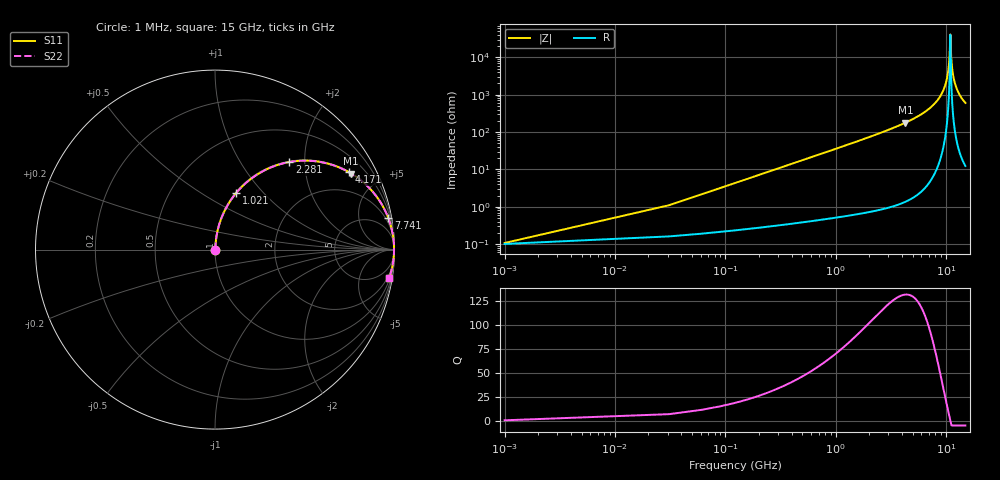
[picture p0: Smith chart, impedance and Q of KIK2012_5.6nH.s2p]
!version-2
!date-01.2022
!Series
# MHz S RI R 50
!Freq ReS11 ImS11 ReS21 ImS21 ReS12 ImS12 ReS22 ImS22
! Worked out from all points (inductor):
!   501 points, 1 MHz to 15 GHz, reference 50 ohm
!   read as one part in series: L = 5.6 nH near 61 MHz
!   highest Q = 131 at 4.291 GHz (marker M1), where L = 6.61 nH
!   self-resonance near 10.95 GHz
!   S11 on the Smith chart (normalised r, x): 1 MHz: 1.00, +0.00; 1.021 GHz: 1.01, +0.72; 2.281 GHz: 1.02, +1.68; 4.171 GHz: 1.03, +3.43; 7.741 GHz: 1, +11; 15 GHz: 1, -12
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1  0.00101 0.000351  0.999 -0.000351  0.999 -0.000351  0.00101 0.000351
91  0.00315 0.0319  0.9969 -0.0319  0.9969 -0.0319  0.00315 0.0319
211  0.00822 0.0735  0.9918 -0.0735  0.9918 -0.0735  0.00822 0.0735
511  0.0349 0.1732  0.9651 -0.1732  0.9651 -0.1732  0.0349 0.1732
1021  0.1196 0.3174  0.8804 -0.3174  0.8804 -0.3174  0.1196 0.3174
2281  0.4139 0.4879  0.5861 -0.4879  0.5861 -0.4879  0.4139 0.4879
2521  0.4676 0.4945  0.5324 -0.4945  0.5324 -0.4945  0.4676 0.4945
4171  0.7449 0.4321  0.2551 -0.4321  0.2551 -0.4321  0.7449 0.4321
4291  0.7591 0.4239  0.2409 -0.4239  0.2409 -0.4239  0.7591 0.4239
5011  0.8306 0.3713  0.1694 -0.3713  0.1694 -0.3713  0.8306 0.3713
7501  0.9589 0.1927  0.0411 -0.1927  0.0411 -0.1927  0.9589 0.1927
7741  0.9652 0.1771  0.0348 -0.1771  0.0348 -0.1771  0.9652 0.1771
9121  0.9887 0.0945  0.0113 -0.0945  0.0113 -0.0945  0.9887 0.0945
10021  0.9956 0.0462  0.00444 -0.0462  0.00444 -0.0462  0.9956 0.0462
10621  0.9974 0.0162  0.00262 -0.0162  0.00262 -0.0162  0.9974 0.0162
10771  0.9975 0.00895  0.00246 -0.00895  0.00246 -0.00895  0.9975 0.00895
10951  0.9976 0.0004  0.0024 -0.0004  0.0024 -0.0004  0.9976 0.0004
11011  0.9976 -0.00242  0.00242 0.00242  0.00242 0.00242  0.9976 -0.00242
11191  0.9974 -0.0108  0.00256 0.0108  0.00256 0.0108  0.9974 -0.0108
11461  0.997 -0.0231  0.00302 0.0231  0.00302 0.0231  0.997 -0.0231
12511  0.9926 -0.0682  0.00738 0.0682  0.00738 0.0682  0.9926 -0.0682
15000  0.9702 -0.16  0.0298 0.16  0.0298 0.16  0.9702 -0.16
